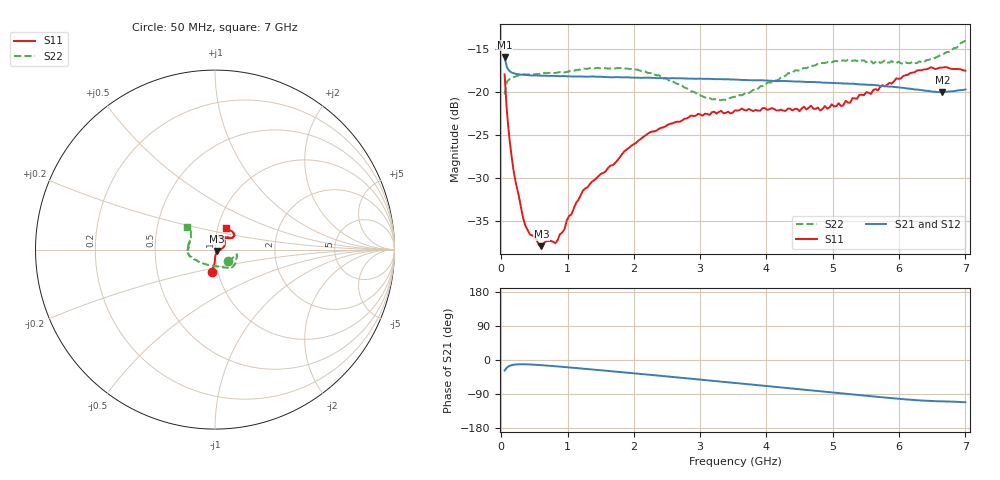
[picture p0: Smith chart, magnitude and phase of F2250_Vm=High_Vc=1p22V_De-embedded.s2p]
! Integrated Device Technology
! Corporate Headquarters
! 6024 Silver Creek Valley Road
! San Jose, CA 95138  USA
! Phone:  1-408-284-8200
! Toll Free:  1-800-223-1366
! Webpage:  http://www.idt.com/
! Timing and RF Division
! 515 Groton Road, Suite 102
! Westford, MA 01886-6024
! Device:  F2250
! Description: Voltage Variable RF Attenuator
! Frequency:  50.0 -  6000.00 MHz
! Package:  3x3 mm Thin QFN Plastic Package: 16 pin
! Ports:  2 RF, 3 DC
!  Pin  1  = GND
!  Pin  2  = NC
!  Pin  3  = RF1  = Port 1
!  Pin  4  = NC
!  Pin  5  = GND
!  Pin  6  = GND
!  Pin  7  = GND
!  Pin  8  = GND
!  Pin  9  = NC
!  Pin 10  = RF2  = Port 2
!  Pin 11  = NC
!  Pin 12  = GND
!  Pin 13  = GND
!  Pin 14  = VCNTRL
!  Pin 15  = VDD
!  Pin 16  = VMODE
! Vcntrl:  1.220 Volts
! Vmode:  +3.300 Volts
! Vdd:  +3.30  Volts
! Current:  1.332 mA
! Data:  The device was measured on a the F2250 evaluation board which has
!  individual transmission lines to the RF pins.  Data was collected
!  using a calibrated network analyzer.  The evaluation board was
!  de-embedded using a TRL calibration technique.
!  The reference plane is the edge of the package pin.
! Misc:  SN 10
!  Action Tracker AT0258
! Date Measured:  2014-11-26
! Date:  2015-10-15  MJV
! Note:
!  Integrated Device Technology supplies this data as a sample of measured
!  data at the package pin for this product.  Your particular data for this
!  product may vary.
!  Data was taken at 25 degrees C.
!  Integrated Device Technology reserves the right to change this data at anytime.
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# GHz S dB R 50
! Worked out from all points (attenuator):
!   201 points, 50 MHz to 7 GHz, reference 50 ohm
!   highest |S21| = -15.92 dB at 50 MHz (marker M1); lowest = -20.0 dB at 6.652 GHz (marker M2)
!   lowest |S11| = -37.9 dB at 606 MHz (marker M3), VSWR 1.03, Z = 51 - j0.788 ohm
!   |S11| at or under -10 dB: start of sweep to end of sweep
!   |S22| runs from -20.9 to -14.0 dB; largest |S21 - S12| = 0.00053
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0.05  -17.93 -98.7  -15.92 -27.9  -15.92 -27.9  -20.27 -41.6
0.08475  -22.28 -91.7  -17.12 -19.9  -17.11 -19.9  -18.79 -20.1
0.15425  -27.42 -89.0  -17.72 -13.7  -17.72 -13.7  -18.42 -12.7
0.189  -29.34 -85.6  -17.81 -12.4  -17.82 -12.4  -18.25 -12.3
0.328  -34.63 -67.9  -17.98 -11.2  -17.99 -11.2  -17.91 -12.9
0.43225  -36.58 -63.8  -18.03 -11.8  -18.05 -11.8  -17.95 -14.2
0.606  -37.94 -37.5  -18.09 -13.6  -18.06 -13.6  -17.82 -19.3
0.6755  -37.37 -34.9  -18.09 -14.5  -18.08 -14.5  -17.79 -20.8
0.8145  -37.60 -19.1  -18.12 -16.4  -18.13 -16.4  -17.77 -24.9
0.9535  -35.97 -22.2  -18.13 -18.5  -18.14 -18.5  -17.71 -28.6
0.98825  -34.92 -20.3  -18.16 -19.0  -18.15 -19.0  -17.66 -29.4
1.2315  -31.45 -6.3  -18.19 -22.7  -18.20 -22.7  -17.28 -34.7
1.857  -26.89 12.5  -18.28 -32.8  -18.27 -32.8  -17.22 -45.3
2.37825  -24.28 26.5  -18.37 -41.3  -18.38 -41.3  -18.03 -55.0
3.07325  -22.51 47.8  -18.45 -53.0  -18.45 -53.0  -20.63 -83.5
3.525  -22.12 61.3  -18.55 -60.6  -18.54 -60.7  -20.54 -115.1
4.7065  -21.94 67.1  -18.82 -80.8  -18.84 -80.8  -16.94 -164.0
5.15825  -21.55 50.3  -19.00 -88.5  -18.98 -88.6  -16.30 -173.1
5.85325  -18.93 35.6  -19.36 -100.1  -19.35 -100.2  -16.57 170.7
6.3745  -17.36 37.7  -19.81 -107.4  -19.79 -107.5  -16.52 153.2
6.6525  -17.15 44.5  -20.00 -109.1  -19.99 -109.3  -15.67 144.2
7  -17.50 62.2  -19.69 -111.5  -19.70 -111.6  -13.98 140.9
